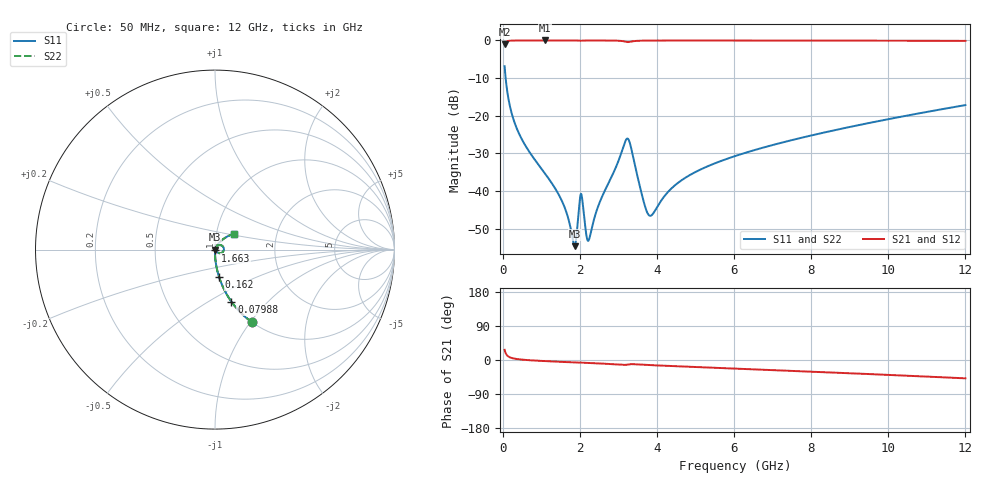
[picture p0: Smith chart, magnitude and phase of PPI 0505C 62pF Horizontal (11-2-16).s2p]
# MHz S MA R 50
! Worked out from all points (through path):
!   1601 points, 50 MHz to 12 GHz, reference 50 ohm
!   highest |S21| = -0.01 dB at 1.103 GHz (marker M1); lowest = -1.0 dB at 50 MHz (marker M2)
!   group delay of S21, straight-line fit = 11.7 ps
!   lowest |S11| = -54.6 dB at 1.865 GHz (marker M3), VSWR 1.00, Z = 50.2 - j0.0724 ohm
!   |S11| at or under -10 dB: 76.66 MHz to end of sweep
!   |S22| runs from -54.6 to -6.8 dB; largest |S21 - S12| = 0
!   S11 on the Smith chart (normalised r, x): 50 MHz: 1.00, -1.02; 79.88 MHz: 1.00, -0.64; 162 MHz: 1.00, -0.31; 1.663 GHz: 1.00, -0.01; 12 GHz: 1.21, +0.22
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50  0.455 -63.1  0.8902 26.9  0.8902 26.9  0.455 -63.1
79.875  0.3044 -72.5  0.9522 17.4  0.9522 17.4  0.3044 -72.5
162.0312  0.155 -81.5  0.9875 8.3  0.9875 8.3  0.155 -81.5
460.7812  0.05289 -87.9  0.998 1.4  0.998 1.4  0.05289 -87.9
1103.094  0.01694 -89.9  0.9989 -2.9  0.9989 -2.9  0.01694 -89.9
1663.25  0.005029 -81.7  0.9987 -5.6  0.9987 -5.6  0.005029 -81.7
1864.906  0.001855 -22.9  0.9981 -6.5  0.9981 -6.5  0.001855 -22.9
1999.344  0.007532 16.6  0.993 -7.2  0.993 -7.2  0.007532 16.6
2044.156  0.008954 -17.9  0.9911 -7.1  0.9911 -7.1  0.008954 -17.9
2171.125  0.00259 -23.8  0.9974 -7.6  0.9974 -7.6  0.00259 -23.8
2238.344  0.002266 18.4  0.9978 -7.9  0.9978 -7.9  0.002266 18.4
2514.688  0.007069 63.9  0.9978 -9.2  0.9978 -9.2  0.007069 63.9
3231.688  0.04982 6.3  0.9524 -12.2  0.9524 -12.2  0.04982 6.3
3321.312  0.03921 -29.1  0.9625 -11.0  0.9625 -11.0  0.03921 -29.1
3747.031  0.00521 -18.8  0.9946 -13.1  0.9946 -13.1  0.00521 -18.8
3859.062  0.004763 13.6  0.9955 -13.6  0.9955 -13.6  0.004763 13.6
4038.312  0.006538 44.0  0.9963 -14.5  0.9963 -14.5  0.006538 44.0
4725.438  0.01489 62.9  0.9971 -17.4  0.9971 -17.4  0.01489 62.9
6025  0.02913 62.7  0.9968 -22.6  0.9968 -22.6  0.02913 62.7
8019.156  0.05498 56.4  0.9953 -30.8  0.9953 -30.8  0.05498 56.4
10013.31  0.09031 48.7  0.9922 -39.3  0.9922 -39.3  0.09031 48.7
12000  0.1385 40.1  0.9861 -48.4  0.9861 -48.4  0.1385 40.1
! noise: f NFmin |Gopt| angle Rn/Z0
50  0.0003696  0.858  0.5212  0.0005565
1372  0.003787  0.66  4.886  0.002125
2701  0.008659  0.701  9.453  0.005634
4031  0.01187  0.6802  14.09  0.007072
5360  0.01151  0.5886  18.51  0.004996
6682  0.01307  0.5603  22.82  0.005145
8012  0.01487  0.5459  27.03  0.005537
9341  0.01677  0.5388  31.11  0.006021
1.067e+04  0.01877  0.5366  35.06  0.006575
1.2e+04  0.02088  0.5384  38.86  0.007204
